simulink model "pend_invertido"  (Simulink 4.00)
settings: Solver=ode45  StartTime=0.0  StopTime=10.0  RelTol=1e-3
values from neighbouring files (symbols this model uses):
  c1 = 0.2254    [Param_pend.m]
  cr = 0.0144    [Param_pend.m]
  g = 9.8    [Param_pend.m]
  Jbar = J0str + mw2*(lw2)^2    (= 0.04317025)    [Param_pend.m]
  l0 = 0.33    [Param_pend.m]
  lc = (mw2*lw2 + m20*lc0)/m2    (= -0.0458067226891)    [Param_pend.m]
  m1 = m10 + mw1    (= 0.238)    [Param_pend.m]
  m2 = m20 + mw2    (= 1.785)    [Param_pend.m]

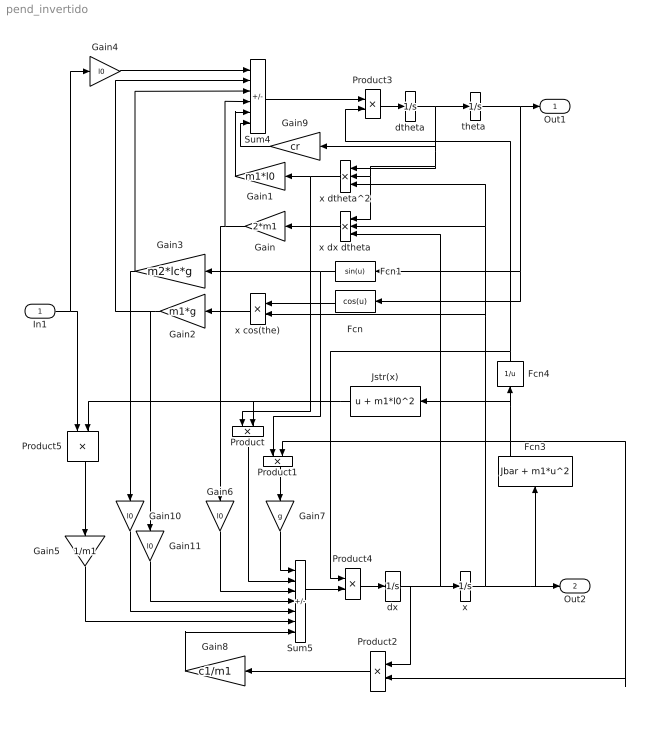
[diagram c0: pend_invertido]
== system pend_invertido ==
  In1 : Inport  Port=1
  Fcn : Fcn  Orientation=left  Expr=cos(u)
  Fcn1 : Fcn  Orientation=left  Expr=sin(u)
  Fcn3 : Fcn  Orientation=up  Expr=Jbar + m1*u^2
  Fcn4 : Fcn  Orientation=up  Expr=1/u
  Gain : Gain  Orientation=left  Gain=2*m1  Multiplication=Element-wise(K.*u)  SaturateOnIntegerOverflow=on
  Gain1 : Gain  Orientation=left  Gain=m1*l0  Multiplication=Element-wise(K.*u)  SaturateOnIntegerOverflow=on
  Gain10 : Gain  Orientation=down  Gain=l0  Multiplication=Element-wise(K.*u)  SaturateOnIntegerOverflow=on
  Gain11 : Gain  Orientation=down  Gain=l0  Multiplication=Element-wise(K.*u)  SaturateOnIntegerOverflow=on
  Gain2 : Gain  Orientation=left  Gain=m1*g  Multiplication=Element-wise(K.*u)  SaturateOnIntegerOverflow=on
  Gain3 : Gain  Orientation=left  Gain=m2*lc*g  Multiplication=Element-wise(K.*u)  SaturateOnIntegerOverflow=on
  Gain4 : Gain  Gain=l0  Multiplication=Element-wise(K.*u)  SaturateOnIntegerOverflow=on
  Gain5 : Gain  Orientation=down  Gain=1/m1  Multiplication=Element-wise(K.*u)  SaturateOnIntegerOverflow=on
  Gain6 : Gain  Orientation=down  Gain=l0  Multiplication=Element-wise(K.*u)  SaturateOnIntegerOverflow=on
  Gain7 : Gain  Orientation=down  Gain=g  Multiplication=Element-wise(K.*u)  SaturateOnIntegerOverflow=on
  Gain8 : Gain  Orientation=left  Gain=c1/m1  Multiplication=Element-wise(K.*u)  SaturateOnIntegerOverflow=on
  Gain9 : Gain  Orientation=left  Gain=cr  Multiplication=Element-wise(K.*u)  SaturateOnIntegerOverflow=on
  Jstr(x) : Fcn  Orientation=left  Expr=u + m1*l0^2
  Product : Product  Orientation=down  Inputs=2  Multiplication=Element-wise(.*)  SaturateOnIntegerOverflow=on
  Product1 : Product  Orientation=down  Inputs=2  Multiplication=Element-wise(.*)  SaturateOnIntegerOverflow=on
  Product2 : Product  Orientation=left  Inputs=2  Multiplication=Element-wise(.*)  SaturateOnIntegerOverflow=on
  Product3 : Product  Inputs=2  Multiplication=Element-wise(.*)  SaturateOnIntegerOverflow=on
  Product4 : Product  Inputs=2  Multiplication=Element-wise(.*)  SaturateOnIntegerOverflow=on
  Product5 : Product  Orientation=down  Inputs=2  Multiplication=Element-wise(.*)  SaturateOnIntegerOverflow=on
  Sum4 : Sum  Inputs=-++---  SaturateOnIntegerOverflow=on
  Sum5 : Sum  Inputs=+++--+-  SaturateOnIntegerOverflow=on
  dtheta : Integrator  ExternalReset=none  InitialConditionSource=internal  InitialCondition=0  LimitOutput=off  UpperSaturationLimit=inf  LowerSaturationLimit=-inf  ShowSaturationPort=off  ShowStatePort=off  AbsoluteTolerance=auto
  dx : Integrator  ExternalReset=none  InitialConditionSource=internal  InitialCondition=0  LimitOutput=off  UpperSaturationLimit=inf  LowerSaturationLimit=-inf  ShowSaturationPort=off  ShowStatePort=off  AbsoluteTolerance=auto
  "theta " : Integrator  ExternalReset=none  InitialConditionSource=internal  InitialCondition=0  LimitOutput=off  UpperSaturationLimit=inf  LowerSaturationLimit=-inf  ShowSaturationPort=off  ShowStatePort=off  AbsoluteTolerance=auto
  x : Integrator  ExternalReset=none  InitialConditionSource=internal  InitialCondition=0  LimitOutput=off  UpperSaturationLimit=inf  LowerSaturationLimit=-inf  ShowSaturationPort=off  ShowStatePort=off  AbsoluteTolerance=auto
  x cos(the) : Product  Orientation=left  Inputs=2  Multiplication=Element-wise(.*)  SaturateOnIntegerOverflow=on
  x dtheta^2 : Product  Orientation=left  Inputs=3  Multiplication=Element-wise(.*)  SaturateOnIntegerOverflow=on
  x dx dtheta : Product  Orientation=left  Inputs=3  Multiplication=Element-wise(.*)  SaturateOnIntegerOverflow=on
  Out1 : Outport  Port=1  InitialOutput=0
  Out2 : Outport  Port=2  InitialOutput=0
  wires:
  x dx dtheta/1 -> Gain/1
  Gain1/1 -> Sum4/5
  x cos(the)/1 -> Gain2/1
  Gain4/1 -> Sum4/1
  x dtheta^2/1 -> Gain1/1, Product/1
  Gain/1 -> Sum4/4, Gain6/1
  Fcn/1 -> x cos(the)/1
  Fcn4/1 -> Product3/2, Product4/1
  Fcn1/1 -> Product1/1, Gain3/1
  Product1/1 -> Gain7/1
  dx/1 -> x/1, x dx dtheta/3, Product2/1
  x/1 -> x dx dtheta/2, x dtheta^2/3, x cos(the)/2, Out2/1, Fcn3/1
  Product4/1 -> dx/1
  Sum5/1 -> Product4/2
  Gain6/1 -> Sum5/3
  Product/1 -> Sum5/2
  Gain7/1 -> Sum5/1
  Gain3/1 -> Sum4/3, Gain10/1
  Gain5/1 -> Sum5/6
  Gain10/1 -> Sum5/5
  Gain2/1 -> Sum4/2, Gain11/1
  Gain11/1 -> Sum5/4
  In1/1 -> Gain4/1, Product5/1
  Jstr(x)/1 -> Product/2, Product5/2
  Product5/1 -> Gain5/1
  Fcn3/1 -> Fcn4/1, Jstr(x)/1, Product1/2, Product2/2
  dtheta/1 -> "theta "/1, x dtheta^2/1, x dtheta^2/2, x dx dtheta/1, Gain9/1
  "theta "/1 -> Fcn/1, Fcn1/1, Out1/1
  Product3/1 -> dtheta/1
  Sum4/1 -> Product3/1
  Product2/1 -> Gain8/1
  Gain8/1 -> Sum5/7
  Gain9/1 -> Sum4/6
